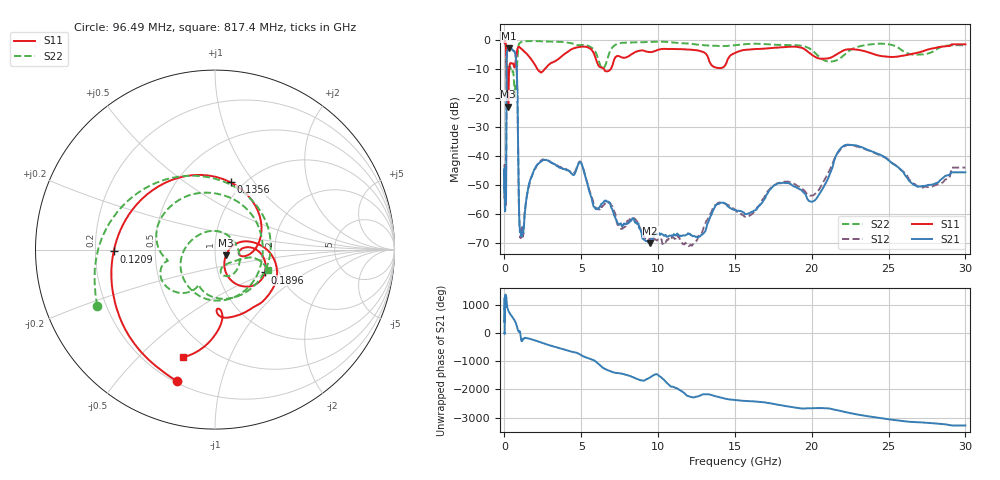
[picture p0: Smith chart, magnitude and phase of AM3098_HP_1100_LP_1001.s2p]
! Date/Time: Thu, Feb 28, 2019 8:44 AM
! Network Analyzer: Agilent Technologies E8364B Rev: A.07.50.67
! Sweep from 0.010 to 30.000 GHz, 1601 Points, Sweep Type: LOG
! Power Supply: 5.023 V, 0.002 A
# Hz S DB R 50
!freq MagS11 AngS11 MagS21 AngS21 MagS12 AngS12 MagS22 AngS22
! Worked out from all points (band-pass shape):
!   1601 points, 10 MHz to 30 GHz, reference 50 ohm
!   highest |S21| = -3.05 dB at 265.1 MHz (marker M1); lowest = -70.3 dB at 9.49 GHz (marker M2)
!   |S21| within 3 dB of the highest: 149.3 MHz to 735.7 MHz (586.5 MHz wide, 133 % of centre)
!   lowest |S11| = -23.2 dB at 247.2 MHz (marker M3), VSWR 1.15, Z = 56.5 - j3.54 ohm
!   |S11| at or under -10 dB: 140.1 MHz to 314.6 MHz (174.5 MHz wide, 76.8 % of centre); 2.118 GHz to 2.666 GHz (548.2 MHz wide, 22.9 % of centre); 6.452 GHz to 6.94 GHz (488.5 MHz wide, 7.3 % of centre)
!   |S22| runs from -19.8 to -0.5 dB; largest |S21 - S12| = 0.012
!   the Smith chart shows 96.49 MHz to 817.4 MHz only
!   S11 on the Smith chart (normalised r, x): 96.49 MHz: 0.21, -0.73; 120.9 MHz: 0.28, -0.01; 135.6 MHz: 0.87, +0.77; 189.6 MHz: 1.69, -0.47; 817.4 MHz: 0.35, -0.69
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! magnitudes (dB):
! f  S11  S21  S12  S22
! 10 MHz  -0.4  -45.0  -44.0  -0.6
! 38.04 MHz  -0.4  -55.6  -57.1  -0.8
! 96.49 MHz  -2.3  -54.0  -55.2  -2.8
! 120.9 MHz  -5.0  -36.2  -35.9  -6.5
! 135.6 MHz  -8.3  -13.9  -13.9  -10.3
! 144.7 MHz  -12.3  -7.4  -7.4  -11.6
! 189.6 MHz  -10.3  -3.7  -3.7  -9.4
! 247.2 MHz  -23.2  -3.1  -3.0  -11.4
! 265.1 MHz  -18.2  -3.0  -3.0  -11.2
! 550.5 MHz  -8.3  -3.8  -3.7  -10.9
! 669.1 MHz  -9.5  -4.4  -4.3  -19.7
! 817.4 MHz  -4.1  -13.1  -13.0  -10.0
! 949.8 MHz  -2.5  -59.4  -59.2  -1.5
! 1.034 GHz  -2.9  -66.3  -68.0  -1.0
! 2.084 GHz  -9.7  -43.6  -43.6  -0.6
! 4.952 GHz  -2.5  -42.3  -42.2  -1.9
! 7.926 GHz  -6.2  -63.4  -63.6  -1.1
! 9.49 GHz  -4.3  -70.3  -68.6  -0.9
! 20.1 GHz  -5.6  -55.8  -53.7  -4.0
! 22.56 GHz  -3.3  -36.4  -36.5  -3.5
! 27.42 GHz  -3.7  -50.4  -50.7  -5.0
! 30 GHz  -1.7  -45.8  -44.1  -2.0
